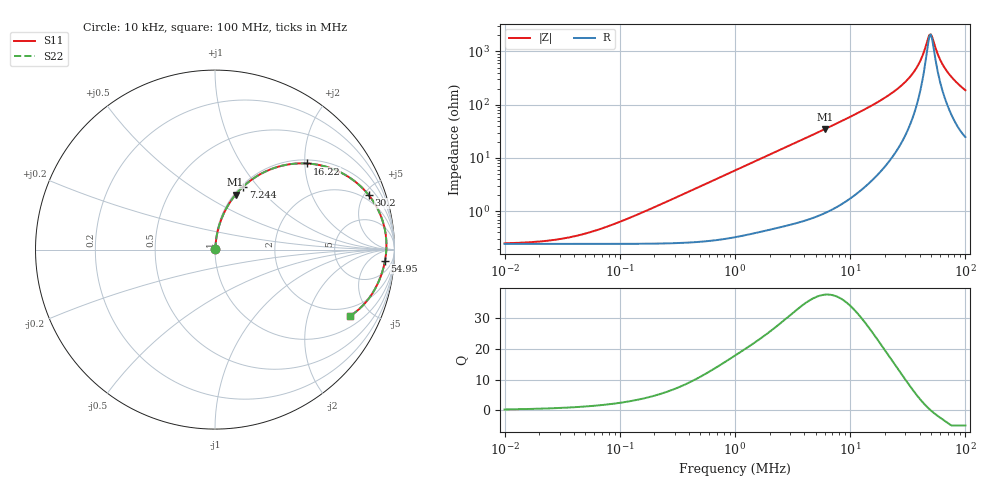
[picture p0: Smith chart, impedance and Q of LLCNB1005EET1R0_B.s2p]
! LLCNB1005EET1R0_B  S-PARAMETER MODEL  ( Standard Model )
! Model Generated by TAIYO YUDEN Corporation (http://www.ty-top.com)
! Version 1.0
! TAIYO YUDEN Control No. 190130
! Copyright(c) 2019 TAIYO YUDEN CO.,LTD. All Rights Reserved.
! Product Description (link to TY-COMPAS)
! https://ds.yuden.co.jp/TYCOMPAS/or/detail?pn=LLCNB1005EET1R0MB&u=M
! Products Name : Inductors
! Characteristics :
!  Inductance : 1.0 [uH] , SRF(min) : - [Hz] , DC Resistance(max) : 300 [mOhm]
!  Rated Current : Saturation  1.0 [A] (dL = 30 [%]), Temp Rise  0.8 [A] (dT = 40 [degC])
!  Case Size : 1.0 x 0.5 / 0.039 x 0.02 [mm/inch] , Thickness : 0.55 / 0.022 [mm/inch]
!  (Conditions: Temperature = 25 [degC] , DC Bias Current = 0 [A])
! External Node Assignments :
!  1  o---GGG---o  2
! GND o---------o GND
! Frequency Range : 10kHz  -  100MHz  [ 402 STEP ]
# MHz S RI R 50
! Freq[MHz].  S11 Real  S11 Imag  S21 Real  S21 Imag  S12 Real  S12 Imag  S22 Real  S22 Imag
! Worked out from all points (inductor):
!   401 points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, 10 kHz to 100 MHz, reference 50 ohm
!   read as one part in series: L = 932 nH near 125.9 kHz
!   highest Q = 37.8 at 6.026 MHz (marker M1), where L = 921 nH
!   self-resonance near 49.81 MHz
!   S11 on the Smith chart (normalised r, x): 10 kHz: 1.00, +0.00; 7.244 MHz: 1.02, +0.84; 16.22 MHz: 1.08, +2.06; 30.2 MHz: 1.54, +5.38; 54.95 MHz: 15, -19; 100 MHz: 1.49, -3.71
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0.01  0.00243 0.000582  0.9976 -0.000582  0.9976 -0.000582  0.00243 0.000582
0.023988  0.00244 0.0014  0.9976 -0.0014  0.9976 -0.0014  0.00244 0.0014
0.046774  0.00244 0.00272  0.9976 -0.00272  0.9976 -0.00272  0.00244 0.00272
0.089125  0.00246 0.00519  0.9975 -0.00519  0.9975 -0.00519  0.00246 0.00519
0.218776  0.00264 0.0127  0.9974 -0.0127  0.9974 -0.0127  0.00264 0.0127
1  0.00659 0.0576  0.9934 -0.0576  0.9934 -0.0576  0.00659 0.0576
2.290868  0.0217 0.1286  0.9783 -0.1286  0.9783 -0.1286  0.0217 0.1286
4.677351  0.0737 0.2479  0.9263 -0.2479  0.9263 -0.2479  0.0737 0.2479
6.025596  0.1149 0.3059  0.8851 -0.3059  0.8851 -0.3059  0.1149 0.3059
7.24436  0.1577 0.3514  0.8423 -0.3514  0.8423 -0.3514  0.1577 0.3514
10.71519  0.296 0.4416  0.704 -0.4416  0.704 -0.4416  0.296 0.4416
16.2181  0.5147 0.4798  0.4853 -0.4798  0.4853 -0.4798  0.5147 0.4798
21.87762  0.6929 0.4336  0.3071 -0.4336  0.3071 -0.4336  0.6929 0.4336
30.19952  0.8564 0.304  0.1436 -0.304  0.1436 -0.304  0.8564 0.304
38.90451  0.9348 0.1574  0.0652 -0.1574  0.0652 -0.1574  0.9348 0.1574
48.97788  0.955 0.0106  0.045 -0.0106  0.045 -0.0106  0.955 0.0106
51.28614  0.9533 -0.0183  0.0467 0.0183  0.0467 0.0183  0.9533 -0.0183
54.95409  0.9475 -0.061  0.0525 0.061  0.0525 0.061  0.9475 -0.061
60.25596  0.9344 -0.1161  0.0656 0.1161  0.0656 0.1161  0.9344 -0.1161
69.1831  0.9039 -0.1953  0.0961 0.1953  0.0961 0.1953  0.9039 -0.1953
83.17638  0.8406 -0.293  0.1594 0.293  0.1594 0.293  0.8406 -0.293
100  0.75 -0.3714  0.25 0.3714  0.25 0.3714  0.75 -0.3714
